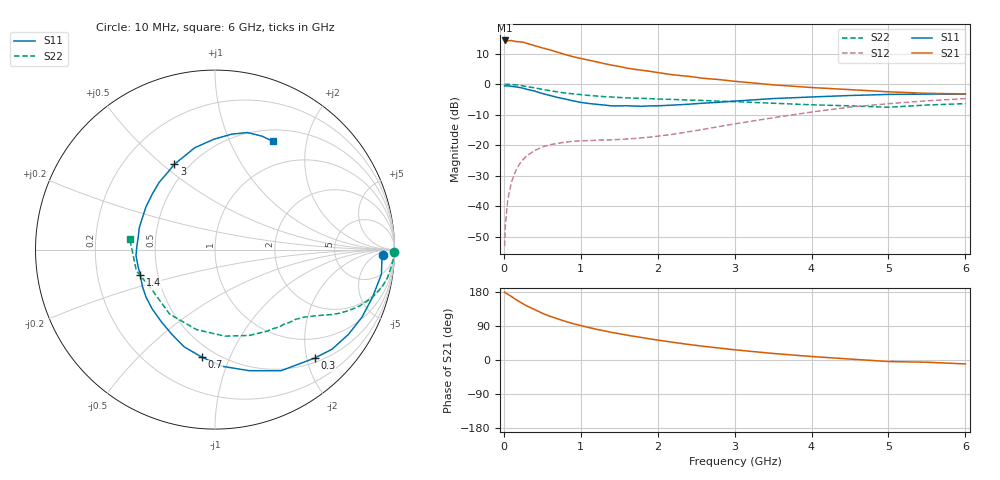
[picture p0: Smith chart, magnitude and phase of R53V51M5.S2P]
! SIEMENS Small Signal Semiconductors
! BFR183
! Si NPN RF Bipolar Junction Transistor in SOT23
! VCE = 3.5 V  IC = 1.5 mA
! Common Emitter S-Parameters:  May  1996
# GHz  S  MA  R  50
!  f  S11  S21  S12  S22
! GHz  MAG  ANG  MAG  ANG  MAG  ANG  MAG  ANG
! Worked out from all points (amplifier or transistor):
!   36 points, 10 MHz to 6 GHz, reference 50 ohm
!   highest |S21| = 14.3 dB at 10 MHz (marker M1)
!   |S21| within 3 dB of that: start of sweep to 586 MHz
!   unconditionally stable (mu >= 1): 1.515 GHz to 2.876 GHz
!   at 250 MHz: K = 0.20, MSG = 19.2 dB, |S12| = -24.8 dB
!   at 1.4 GHz: K = 0.96, MSG = 12.3 dB, |S12| = -18.3 dB
!   at 6 GHz: K = 0.92, MSG = 0.8 dB, |S12| = -4.8 dB
!   S11 on the Smith chart (normalised r, x): 10 MHz: 25, -11; 300 MHz: 0.58, -2.15; 700 MHz: 0.42, -0.79; 1.4 GHz: 0.40, -0.14; 3 GHz: 0.42, +0.55; 6 GHz: 0.65, +1.46
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0.01  0.9349 -1.7  5.192 179.1  0.0022 88.6  0.9988 -0.7
0.02  0.9319 -3.4  5.154 177.3  0.0048 91.1  0.9878 -1.2
0.05  0.9372 -8.4  5.139 173.7  0.0125 85.8  0.9946 -3.2
0.1  0.9173 -16.6  5.171 167.4  0.0249 80.4  0.9841 -6.2
0.15  0.9014 -24.6  5.002 160.3  0.0367 75.6  0.9727 -9.5
0.25  0.8562 -40.4  4.862 148.2  0.0578 66.7  0.9337 -14.9
0.3  0.821 -47.4  4.645 142.5  0.0669 63.6  0.9111 -17.4
0.4  0.7683 -61.5  4.268 133.2  0.0815 56.9  0.8661 -21.2
0.5  0.7007 -74.3  3.923 123.3  0.0926 51.4  0.8203 -24.4
0.6  0.6511 -86.5  3.637 115.4  0.1013 47.0  0.7787 -27.1
0.7  0.6038 -97.0  3.328 108.5  0.1067 43.8  0.7444 -29.1
0.8  0.568 -107.7  3.043 102.0  0.1115 41.2  0.7135 -30.7
0.9  0.5303 -116.8  2.812 96.1  0.1155 39.4  0.6917 -32.0
1.1  0.4813 -136.7  2.477 86.0  0.1183 37.9  0.6527 -34.7
1.4  0.4397 -161.0  2.045 72.9  0.1216 38.6  0.6141 -38.3
1.9  0.4388 164.6  1.619 55.6  0.1352 45.7  0.5769 -45.2
2.2  0.4523 148.3  1.418 46.7  0.1503 50.1  0.5607 -50.1
3  0.5263 115.5  1.112 26.9  0.2225 55.2  0.5158 -68.0
3.5  0.5788 101.2  0.972 17.3  0.2803 52.8  0.4853 -83.5
4.5  0.6498 81.8  0.811 2.5  0.4198 40.6  0.4395 -125.1
5.5  0.6842 67.4  0.705 -5.9  0.5317 24.9  0.4537 -164.9
6  0.6836 62.0  0.69 -10.4  0.5779 15.4  0.4782 173.0
